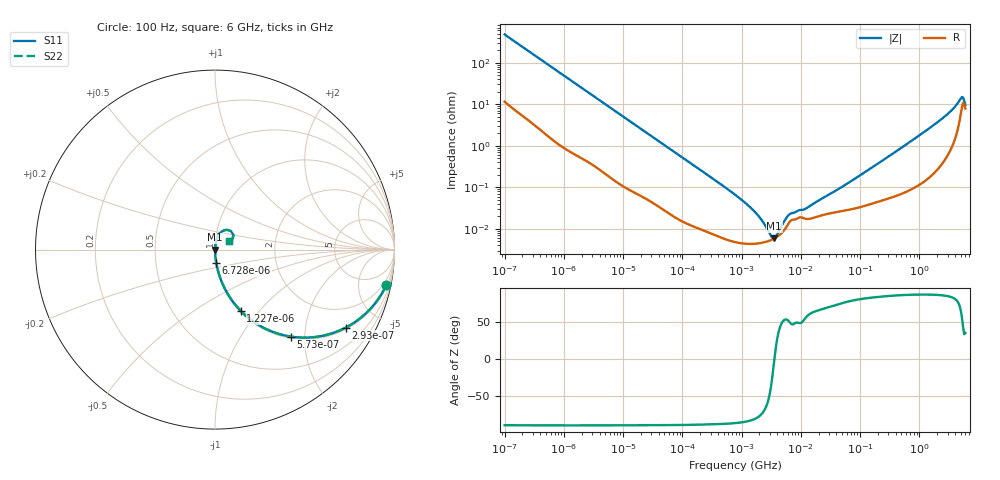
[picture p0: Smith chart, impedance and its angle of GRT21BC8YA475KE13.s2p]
!Murata Part Number: GRT21BC8YA475KE13
!These Parameters are Measured in Series Mode Connection
!Data Generated on Jun 19, 2026
!  o--ll--o
!Port1  Port2
!  o------o
!Operation Temp=25[degC], DC Bias Voltage=0[V]
!Freq. Start=100[Hz] Stop=6[GHz] 401[Steps]
# Hz S RI R 50
!Freq.(Hz) S11(Real) S11(Imag) S21(Real) S21(Imag) S12(Real) S12(Imag) S22(Real) S22(Imag)
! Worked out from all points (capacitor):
!   401 points, 100 Hz to 6 GHz, reference 50 ohm
!   read as one part in series: C = 3.31 uF near 109 Hz
!   lowest |Z| = 5.87 mohm at 3.55 MHz (marker M1)
!   series resonance near 3.586 MHz, so ESL is about 590 pH
!   S11 on the Smith chart (normalised r, x): 100 Hz: 1.23, -9.57; 293 Hz: 1.07, -3.31; 573 Hz: 1.03, -1.71; 1.227 kHz: 1.01, -0.80; 6.728 kHz: 1.00, -0.15; 6 GHz: 1.16, +0.11
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100  0.9538 -0.1982  0.0462 0.1982  0.0462 0.1982  0.9538 -0.1982
179  0.8735 -0.3215  0.1265 0.3215  0.1265 0.3215  0.8735 -0.3215
293  0.7289 -0.4342  0.2711 0.4342  0.2711 0.4342  0.7289 -0.4342
573  0.4229 -0.4848  0.5771 0.4848  0.5771 0.4848  0.4229 -0.4848
1227  0.1433 -0.3413  0.8567 0.3413  0.8567 0.3413  0.1433 -0.3413
2008  0.0615 -0.2303  0.9385 0.2303  0.9385 0.2303  0.0615 -0.2303
6728  0.00709 -0.0743  0.9929 0.0743  0.9929 0.0743  0.00709 -0.0743
40335  0.000502 -0.0128  0.9995 0.0128  0.9995 0.0128  0.000502 -0.0128
774597  4.84e-05 -0.000665  1 0.000665  1 0.000665  4.84e-05 -0.000665
1585629  4.37e-05 -0.000275  1 0.000275  1 0.000275  4.37e-05 -0.000275
2713602  4.98e-05 -8.57e-05  1 8.57e-05  1 8.57e-05  4.98e-05 -8.57e-05
3549919  5.86e-05 -3e-06  0.9999 3e-06  0.9999 3e-06  5.86e-05 -3e-06
4440638  7.27e-05 6.63e-05  0.9999 -6.63e-05  0.9999 -6.63e-05  7.27e-05 6.63e-05
6644369  0.000154 0.000173  0.9998 -0.000173  0.9998 -0.000173  0.000154 0.000173
1.189169e7  0.000175 0.000247  0.9998 -0.000247  0.9998 -0.000247  0.000175 0.000247
1.555665e7  0.000181 0.000342  0.9998 -0.000342  0.9998 -0.000342  0.000181 0.000342
5.960426e7  0.000283 0.00117  0.9997 -0.00117  0.9997 -0.00117  0.000283 0.00117
3.124326e8  0.000578 0.00567  0.9994 -0.00567  0.9994 -0.00567  0.000578 0.00567
2.240541e9  0.00484 0.0408  0.9952 -0.0408  0.9952 -0.0408  0.00484 0.0408
3.505958e9  0.0137 0.0692  0.9863 -0.0692  0.9863 -0.0692  0.0137 0.0692
5.016141e9  0.068 0.1102  0.932 -0.1102  0.932 -0.1102  0.068 0.1102
6e9  0.0753 0.0469  0.9247 -0.0469  0.9247 -0.0469  0.0753 0.0469
